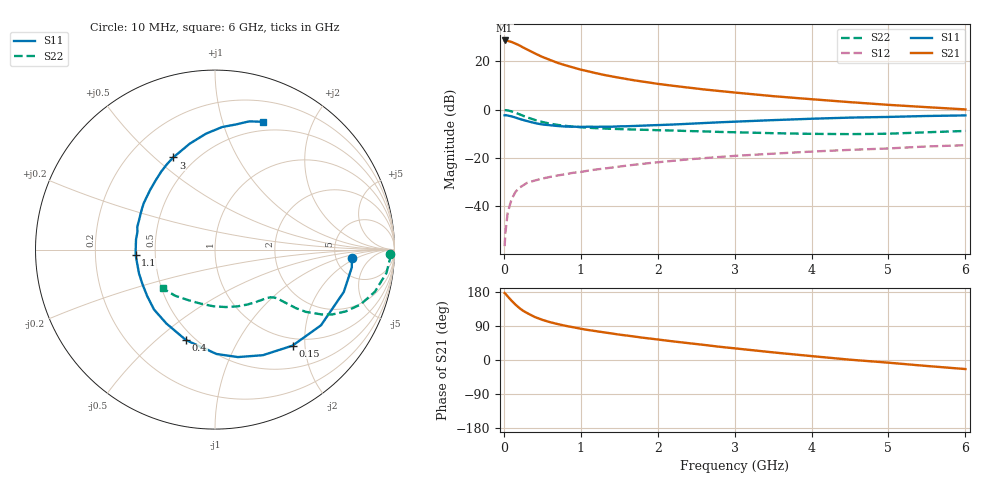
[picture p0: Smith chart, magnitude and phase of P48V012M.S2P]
! SIEMENS Small Signal Semiconductors
! BFP182
! Si NPN RF Bipolar Junction Transistor in SOT143
! VCE = 8 V  IC = 12 mA
! Common Emitter S-Parameters:  March  1996
# GHz  S  MA  R  50
!  f  S11  S21  S12  S22
! GHz  MAG  ANG  MAG  ANG  MAG  ANG  MAG  ANG
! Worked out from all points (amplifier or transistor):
!   36 points, 10 MHz to 6 GHz, reference 50 ohm
!   highest |S21| = 28.6 dB at 10 MHz (marker M1)
!   |S21| within 3 dB of that: start of sweep to 257.4 MHz
!   unconditionally stable (mu >= 1): 1.185 GHz to 5.487 GHz
!   at 250 MHz: K = 0.34, MSG = 28.5 dB, |S12| = -31.3 dB
!   at 1.4 GHz: K = 1.07, MAG = 17.3 dB, |S12| = -24.0 dB
!   at 6 GHz: K = 0.96, MSG = 7.4 dB, |S12| = -14.7 dB
!   S11 on the Smith chart (normalised r, x): 10 MHz: 7.12, -1.55; 150 MHz: 0.87, -1.76; 400 MHz: 0.45, -0.63; 1.1 GHz: 0.39, -0.03; 3 GHz: 0.38, +0.58; 6 GHz: 0.40, +1.36
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0.01  0.7636 -3.4  26.97 176.9  0.0015 85.8  0.9773 -1.4
0.02  0.7687 -7.4  26.91 175.1  0.0028 81.5  0.976 -3.1
0.05  0.7554 -18.2  26.48 167.8  0.0074 82.6  0.9643 -7.7
0.1  0.7257 -35.5  25.11 156.5  0.0139 72.9  0.921 -14.8
0.15  0.6876 -51.1  23.25 146.4  0.0197 65.8  0.8662 -20.7
0.2  0.646 -65.6  21.41 137.5  0.0241 61.4  0.8057 -25.3
0.25  0.6122 -78.0  19.36 130.0  0.0271 56.7  0.7472 -28.9
0.3  0.5815 -89.2  17.64 124.2  0.0305 54.0  0.6951 -31.3
0.4  0.5294 -107.8  14.65 113.7  0.0341 49.8  0.6144 -34.4
0.5  0.4929 -123.3  12.32 106.0  0.0375 47.0  0.5555 -35.9
0.6  0.4764 -135.5  10.68 99.9  0.0406 46.6  0.5136 -36.6
0.7  0.4581 -145.5  9.262 94.8  0.0435 46.0  0.4834 -37.2
0.9  0.4438 -162.5  7.455 86.5  0.0494 45.7  0.4456 -38.0
1.1  0.4431 -176.2  6.179 79.0  0.0548 46.5  0.4223 -39.2
1.5  0.4511 163.6  4.565 67.0  0.0664 46.1  0.3963 -42.9
1.8  0.4662 150.8  3.815 59.0  0.0754 45.6  0.384 -46.6
2.2  0.4922 136.9  3.114 49.1  0.0874 43.5  0.3701 -52.8
3  0.5637 114.4  2.26 30.8  0.1105 37.9  0.3408 -68.0
3.5  0.6068 103.4  1.901 20.1  0.1228 33.9  0.3258 -79.3
4.5  0.6843 86.6  1.429 0.8  0.1473 26.1  0.3115 -105.1
5.5  0.7393 75.1  1.125 -15.8  0.1732 19.0  0.3403 -131.1
6  0.7599 69.6  1.011 -23.9  0.1836 14.4  0.3625 -143.7
